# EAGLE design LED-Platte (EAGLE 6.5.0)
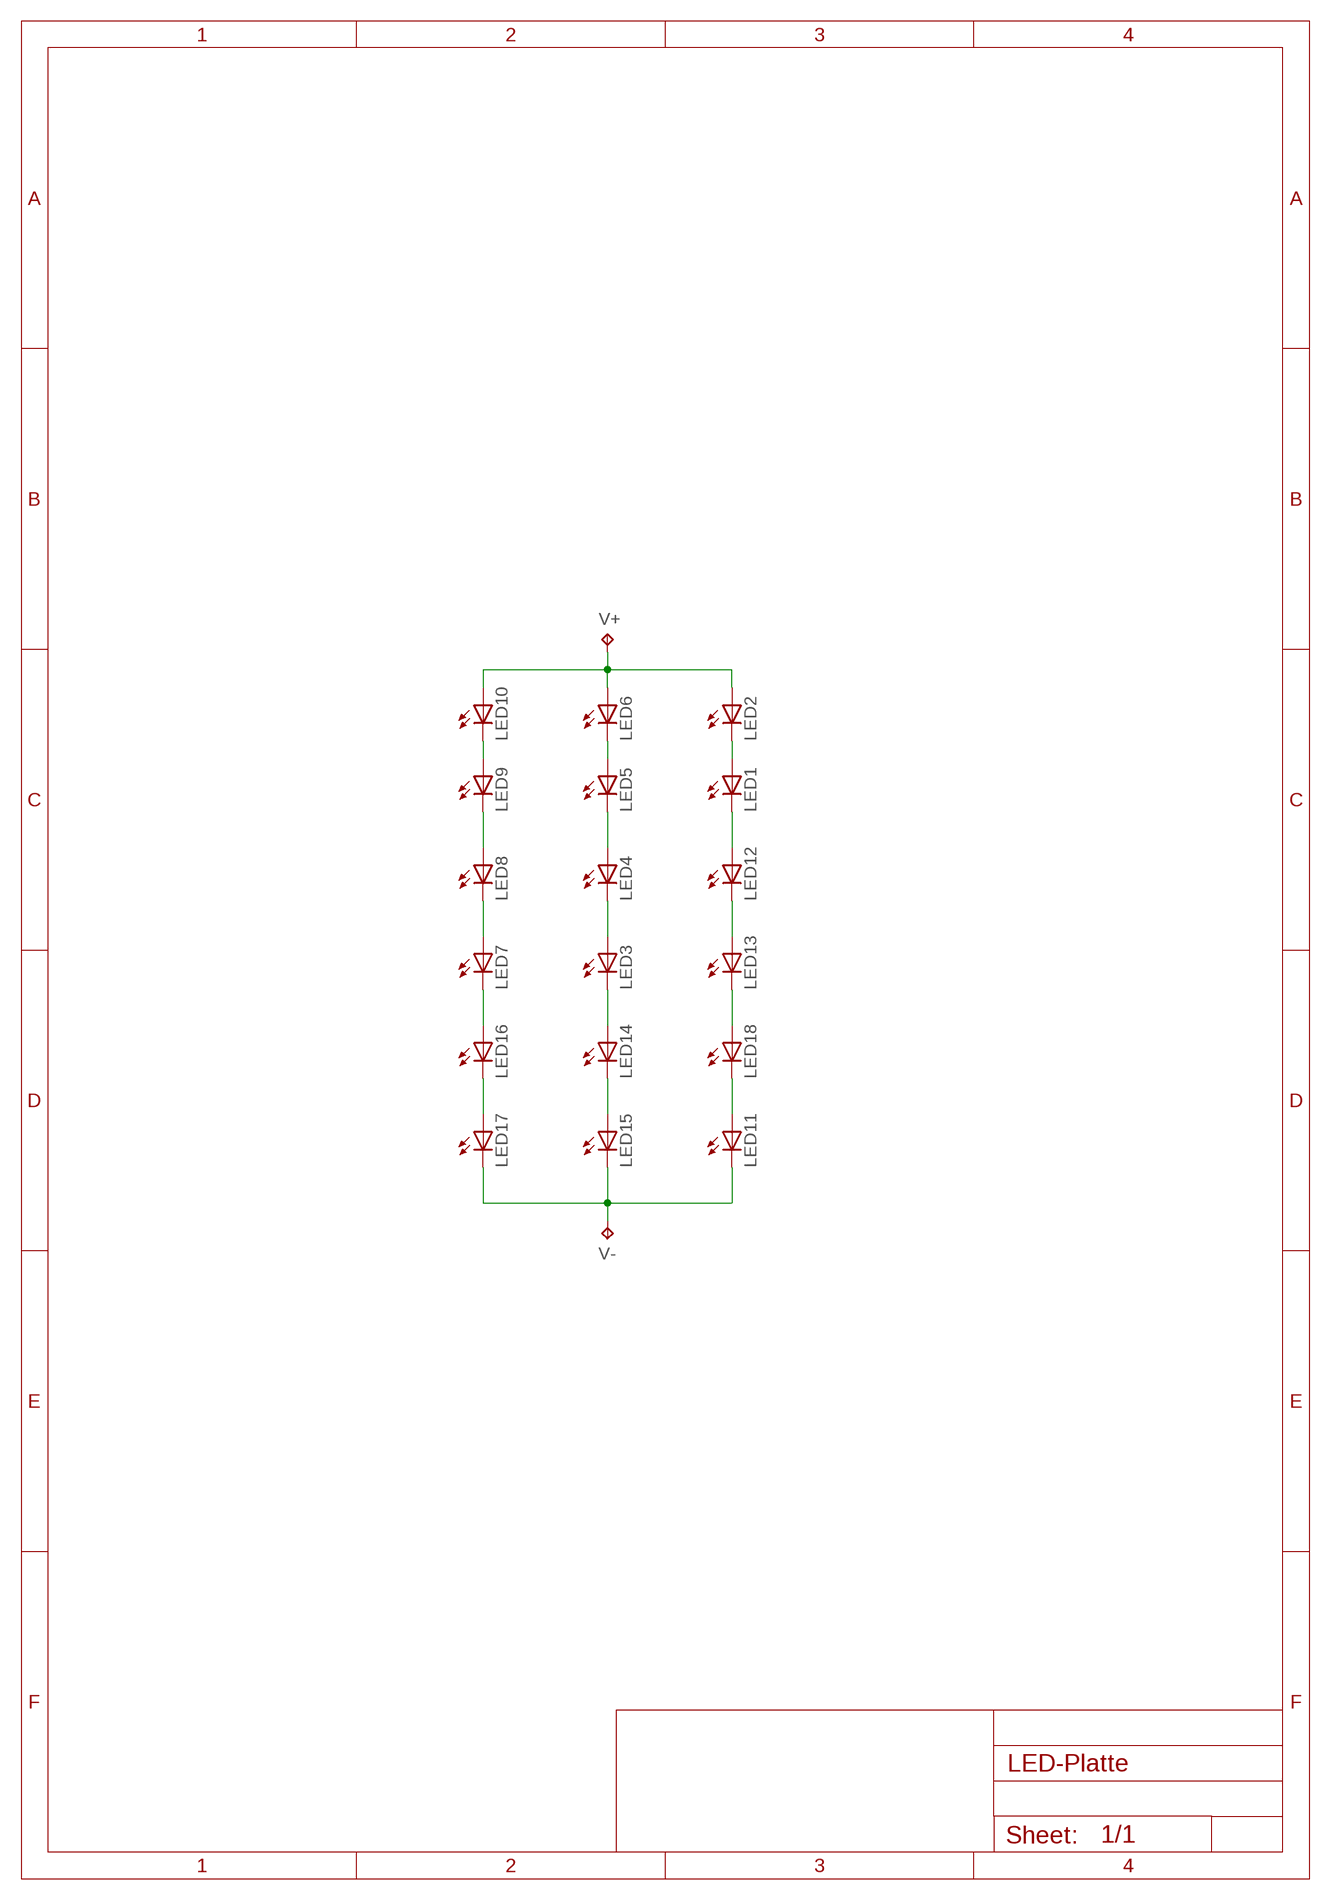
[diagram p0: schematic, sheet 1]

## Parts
LED1  LED-5730  [LED5730]
LED2  LED-5730  [LED5730]
LED3  LED-5730  [LED5730]
LED4  LED-5730  [LED5730]
LED5  LED-5730  [LED5730]
LED6  LED-5730  [LED5730]
LED7  LED-5730  [LED5730]
LED8  LED-5730  [LED5730]
LED9  LED-5730  [LED5730]
LED10  LED-5730  [LED5730]
LED11  LED-5730  [LED5730]
LED12  LED-5730  [LED5730]
LED13  LED-5730  [LED5730]
LED14  LED-5730  [LED5730]
LED15  LED-5730  [LED5730]
LED16  LED-5730  [LED5730]
LED17  LED-5730  [LED5730]
LED18  LED-5730  [LED5730]
V+  TPB2,54  [B2,54]
V-  TPB2,54  [B2,54]

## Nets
N$1: LED8.1(A) LED8.2(A) LED9.3(C)
N$2: LED7.1(A) LED7.2(A) LED8.3(C)
N$3: LED9.1(A) LED9.2(A) LED10.3(C)
N$4: LED7.3(C) LED16.1(A) LED16.2(A)
N$5: LED16.3(C) LED17.1(A) LED17.2(A)
N$6: LED5.1(A) LED5.2(A) LED6.3(C)
N$7: LED4.1(A) LED4.2(A) LED5.3(C)
N$8: LED3.1(A) LED3.2(A) LED4.3(C)
N$9: LED3.3(C) LED14.1(A) LED14.2(A)
N$10: LED14.3(C) LED15.1(A) LED15.2(A)
N$11: LED1.1(A) LED1.2(A) LED2.3(C)
N$12: LED1.3(C) LED12.1(A) LED12.2(A)
N$13: LED12.3(C) LED13.1(A) LED13.2(A)
N$14: LED13.3(C) LED18.1(A) LED18.2(A)
N$15: LED11.1(A) LED11.2(A) LED18.3(C)
N$16: LED11.3(C) LED15.3(C) LED17.3(C) V-.TP
N$17: LED2.1(A) LED2.2(A) LED6.1(A) LED6.2(A) LED10.1(A) LED10.2(A) V+.TP

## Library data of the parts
LED1-LED18 = Brunner:LED
V+ V- = testpad:TP: Test pad

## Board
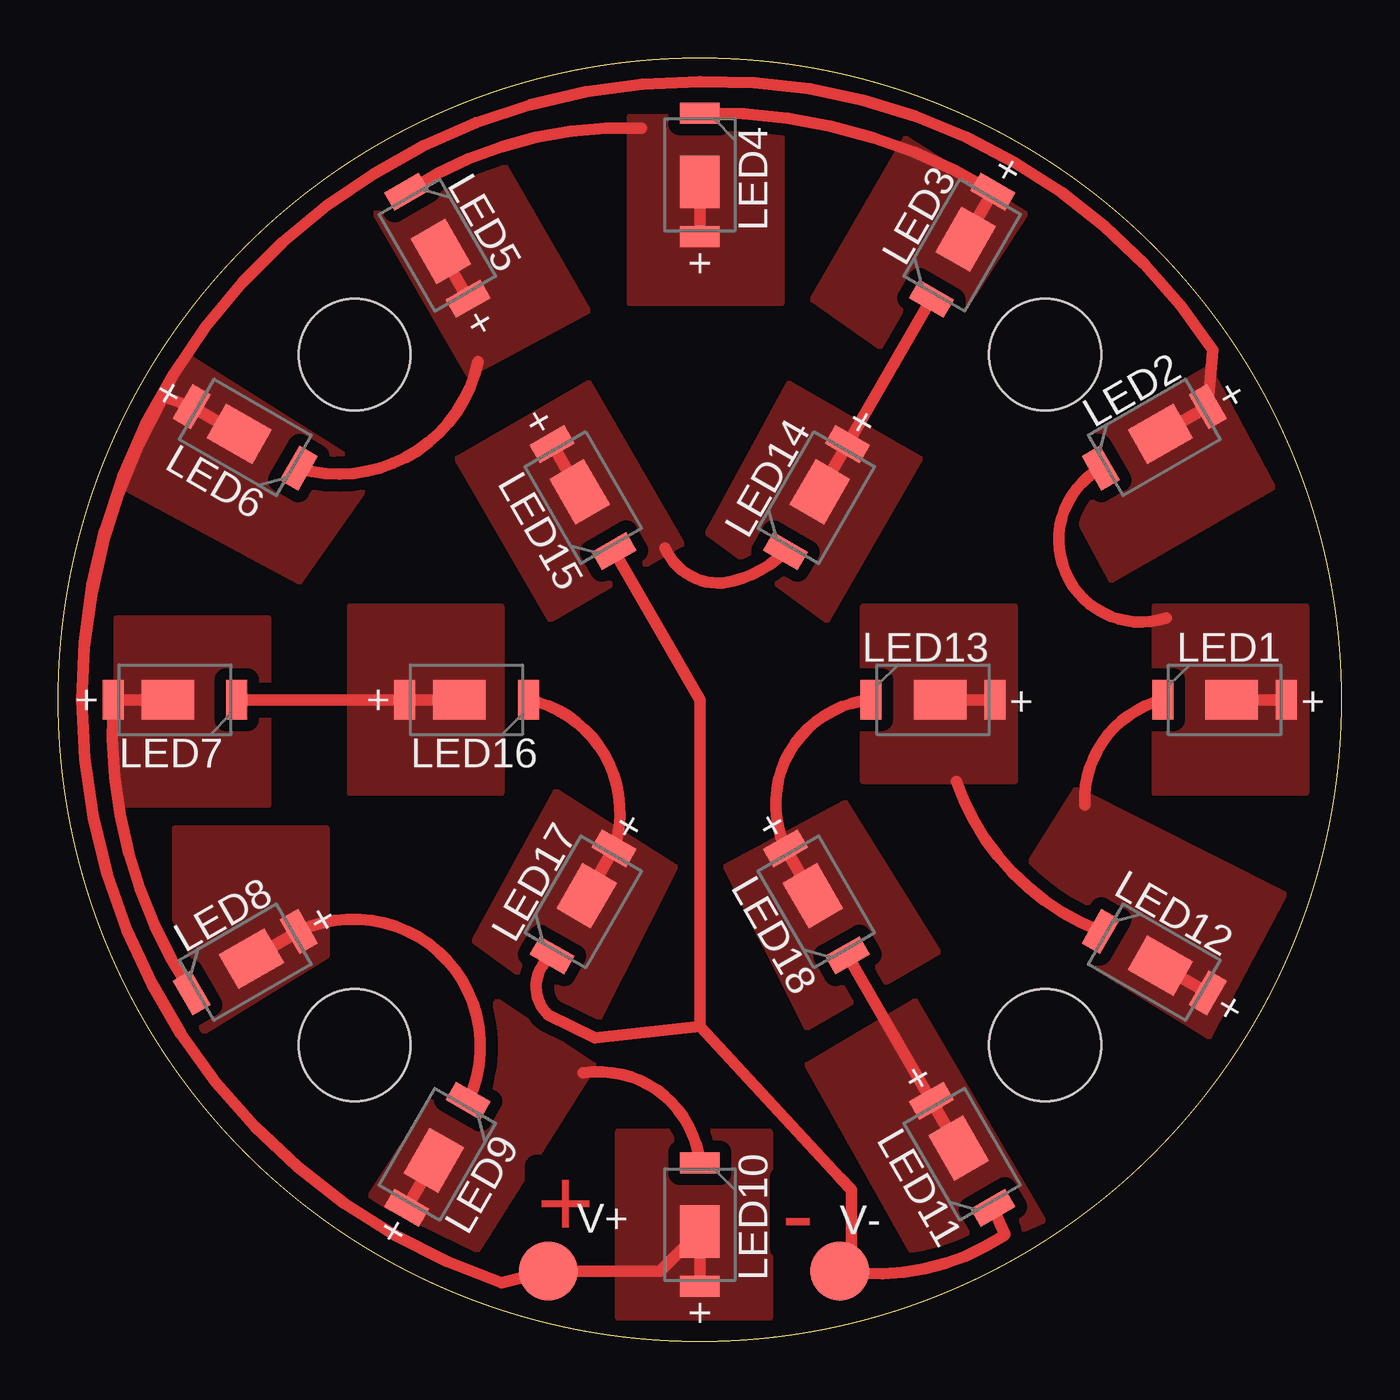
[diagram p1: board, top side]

Size 55 x 55 mm. Coordinates in mm from the lower left corner, seen from the top.
Outline: circle at 27.5,27.5 radius 27.5
Copper layers (1*16): Top 0.035mm / dielectric 1.5mm / Bottom 0.035mm
Design rules "default *": minimum track width 0.25mm, minimum drill 0.5mm, track to track 0.3mm, track to pad 0.3mm, pad to pad 0.3mm, via to via 0.3mm, smd to smd 8mil, copper to edge 0.5mm, drill to drill 0.3mm, minimum pad ring 10mil, minimum via ring 8mil, stop-mask expansion 4mil, vias tented up to drill 0mil, thermal gap 10mil
Holes 4.8 mm at 12.7,12.7 12.7,42.3 42.3,42.3 42.3,12.7

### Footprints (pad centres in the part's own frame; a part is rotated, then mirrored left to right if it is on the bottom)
LED5730 = smd 0.9 x 1.7: 1 -2.65,0; 3 2.65,0 | smd 2.25 x 1.7: 2 -0.3,0
B2,54 = smd 2.54 x 2.54: TP 0,0

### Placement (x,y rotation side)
LED1  50,27.5 180 top
LED2  46.99,38.75 210 top
LED3  38.75,46.99 240 top
LED4  27.5,50 90 top
LED5  16.25,46.99 120 top
LED6  8.01,38.75 330 top
LED7  5,27.5 0 top
LED8  8.01,16.25 210 top
LED9  16.25,8.01 60 top
LED10  27.5,5 90 top
LED11  38.75,8.01 300 top
LED12  46.99,16.25 150 top
LED13  37.5,27.5 180 top
LED14  32.5,36.16 240 top
LED15  22.5,36.16 300 top
LED16  17.5,27.5 0 top
LED17  22.5,18.84 240 top
LED18  32.5,18.84 300 top
U$1  [A4P-LOC]  not placed on the board
V+  21,3 0 top
V-  33.5,3 0 top

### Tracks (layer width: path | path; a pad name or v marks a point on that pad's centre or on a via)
N$1
  Top 0.5: LED8.2 LED8.1 arc-141 LED9.3
  pour Top (isolate 0.5, no thermals): 5,12.5 5,22 11.5,22 11.5,16.5
N$2
  Top 0.5: LED7.2 LED7.1 arc37 LED8.3
  pour Top (isolate 0.5, no thermals): 2.5,23 2.5,31 9,31 9,23
N$3
  Top 0.5: LED9.2 LED9.1 | LED10.3 arc93 22.5,11.5
  pour Top (isolate 0.5, no thermals): 22.96,11.83 17.96,3.9 13.33,6.15 18.83,14.58
N$4
  Top 0.5: LED7.3 LED16.1 LED16.2
  pour Top (isolate 0.5, no thermals): 12.5,23.5 12.5,31.5 19,31.5 19,23.5
N$5
  Top 0.5: LED17.2 LED17.1 arc97 LED16.3
  pour Top (isolate 0.5, no thermals): 26.46,20.33 22.96,13.4 17.83,17.15 21.33,23.58
N$6
  Top 0.5: LED5.2 LED5.1 | LED6.3 arc94 18,42
  pour Top (isolate 0.5, no thermals): 17.6,41.42 13.6,48.35 18.73,51.1 22.73,44.17
N$7
  Top 0.5: LED4.2 LED4.1 | LED5.3 arc-36 25,52
  pour Top (isolate 0.5, no thermals): 24.5,44.5 24.5,52.5 31,52.5 31,44.5
N$8
  Top 0.5: LED3.2 LED3.1 arc33 LED4.3
  pour Top (isolate 0.5, no thermals): 41.46,48.33 36.96,41.4 32.33,44.65 36.33,51.58
N$9
  Top 0.5: LED14.2 LED14.1 LED3.3
  pour Top (isolate 0.5, no thermals): 36.96,37.83 32.96,30.9 27.83,34.65 31.33,41.08
N$10
  Top 0.5: LED15.1 LED15.2 | LED14.3 arc-36 28.5,32.5 arc-69 26,34
  pour Top (isolate 0.5, no thermals): 21.1,30.92 17.1,37.85 22.73,41.1 26.73,34.17
N$11
  Top 0.5: LED1.2 LED1.1 | LED2.3 arc168 47.5,31
  pour Top (isolate 0.5, no thermals): 47,23.5 47,31.5 53.5,31.5 53.5,23.5
N$12
  Top 0.5: LED12.2 LED12.1 | LED1.3 arc78 44,23
  pour Top (isolate 0.5, no thermals): 49.33,13.04 40.4,18.54 43.65,23.67 52.58,19.17
N$13
  Top 0.5: LED13.2 LED13.1 | LED12.3 arc-49 38.5,24
  pour Top (isolate 0.5, no thermals): 34.5,24 34.5,31.5 41,31.5 41,24
N$14
  Top 0.5: LED18.2 LED18.1 arc-110 LED13.3
  pour Top (isolate 0.5, no thermals): 32.1,13.42 28.6,20.35 33.73,23.1 37.73,16.67
N$15
  Top 0.5: LED11.2 LED11.1 LED18.3
  pour Top (isolate 0.5, no thermals): 37.1,2.92 32.1,11.85 36.73,14.6 42.23,5.17
N$16
  Top 0.5: LED15.3 27.5,27.5 27.5,13.5 | LED11.3 40.58,4.57 40.5,4.5 arc-42 V-.TP 34,3.5 34,6.5 33.5,7 27.5,13.5 | LED17.3 arc100 21,14 23,13 27.5,13.5
N$17
  Top 0.5: 1,27.5 arc-90 27.5,54 arc-58 49.5,42.5 LED2.1 LED2.2 | 1,27.5 arc71 19,2.5 V+.TP 25.8,3 LED10.2 LED10.1 | LED6.2 LED6.1 4.5,40.5 arc29 1,27.5
  pour Top (isolate 0.5, no thermals): 10.33,32.54 2.9,36.54 5.65,42.17 13.58,37.17
  pour Top (isolate 0.5, no thermals): 24,1 24,9 30.5,9 30.5,1
  pour Top (isolate 0.5, no thermals): 52.08,36.6 45.15,32.6 42.4,37.73 49.33,41.73

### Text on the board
Top: + | -
tStop: + | -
